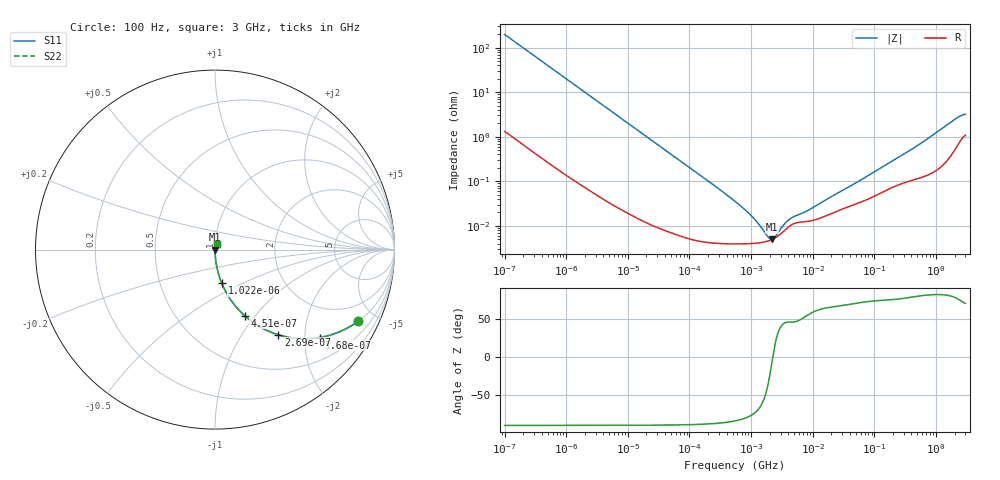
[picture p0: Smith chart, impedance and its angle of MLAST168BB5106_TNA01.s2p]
! MLAST168BB5106_TNA01  S-PARAMETER MODEL  ( Standard Model )
! Model Generated by TAIYO YUDEN Corporation (http://www.ty-top.com)
! Version 1.0
! TAIYO YUDEN Control No. 220601
! Copyright(c) 2015 TAIYO YUDEN CO.,LTD. All Rights Reserved.
! Product Description (link to TY-COMPAS)
! https://ds.yuden.co.jp/TYCOMPAS/or/detail?pn=MLAST168BB5106MTNA01&u=M
! Products Name : Multilayer Ceramic Capacitors
! Characteristics :
!  Capacitance : 10 [uF] , Rated Voltage : 25 [V] , TCC : X5R
!  Case Size : 1.6 x 0.8 / 0.063 x 0.031 [mm/inch] , Thickness : 0.8 / 0.031 [mm/inch]
!  (Conditions: Temperature = 25 [degC] , DC Bias Voltage = 0 [V])
! External Node Assignments :
!  1  o---| |---o  2
! GND o---------o GND
! Frequency Range : 100Hz  -  3GHz  [ 401 STEP ]
# MHZ S RI R 50
! Freq[MHz].  S11 Real  S11 Imag  S21 Real  S21 Imag  S12 Real  S12 Imag  S22 Real  S22 Imag
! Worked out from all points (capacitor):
!   401 points, 100 Hz to 3 GHz, reference 50 ohm
!   read as one part in series: C = 8.04 uF near 109 Hz
!   lowest |Z| = 4.93 mohm at 2.171 MHz (marker M1)
!   series resonance near 2.244 MHz, so ESL is about 630 pH
!   S11 on the Smith chart (normalised r, x): 100 Hz: 1.03, -3.96; 168 Hz: 1.02, -2.37; 269 Hz: 1.01, -1.48; 451 Hz: 1.01, -0.88; 1.022 kHz: 1.00, -0.39; 3 GHz: 1.02, +0.06
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0.0001  0.7949 -0.4005  0.2051 0.4005  0.2051 0.4005  0.7949 -0.4005
0.000119  0.7339 -0.4386  0.2661 0.4386  0.2661 0.4386  0.7339 -0.4386
0.000168  0.5828 -0.4898  0.4172 0.4898  0.4172 0.4898  0.5828 -0.4898
0.000269  0.3538 -0.4748  0.6462 0.4748  0.6462 0.4748  0.3538 -0.4748
0.000451  0.1648 -0.3677  0.8352 0.3677  0.8352 0.3677  0.1648 -0.3677
0.000664  0.0842 -0.2743  0.9158 0.2743  0.9158 0.2743  0.0842 -0.2743
0.001022  0.038 -0.1878  0.962 0.1878  0.962 0.1878  0.038 -0.1878
0.001788  0.0132 -0.1104  0.9868 0.1104  0.9868 0.1104  0.0132 -0.1104
0.005476  0.00165 -0.0367  0.9983 0.0367  0.9983 0.0367  0.00165 -0.0367
0.031977  0.000128 -0.00635  0.9999 0.00635  0.9999 0.00635  0.000128 -0.00635
0.547723  3.93e-05 -0.000353  1 0.000353  1 0.000353  3.93e-05 -0.000353
0.87939  3.96e-05 -0.000198  1 0.000198  1 0.000198  3.96e-05 -0.000198
1.411895  4.17e-05 -8.89e-05  1 8.89e-05  1 8.89e-05  4.17e-05 -8.89e-05
2.171352  4.89e-05 -6.06e-06  1 6.06e-06  1 6.06e-06  4.89e-05 -6.06e-06
3.198641  7.05e-05 6.39e-05  0.9999 -6.39e-05  0.9999 -6.39e-05  7.05e-05 6.39e-05
4.513443  0.000105 0.000108  0.9999 -0.000108  0.9999 -0.000108  0.000105 0.000108
9.794414  0.000131 0.000213  0.9999 -0.000213  0.9999 -0.000213  0.000131 0.000213
175.1444  0.000682 0.0025  0.9993 -0.0025  0.9993 -0.0025  0.000682 0.0025
536.3016  0.00122 0.00664  0.9988 -0.00664  0.9988 -0.00664  0.00122 0.00664
2126.076  0.00625 0.0249  0.9938 -0.0249  0.9938 -0.0249  0.00625 0.0249
2525.516  0.00901 0.028  0.991 -0.028  0.991 -0.028  0.00901 0.028
3000  0.0115 0.0295  0.9885 -0.0295  0.9885 -0.0295  0.0115 0.0295
